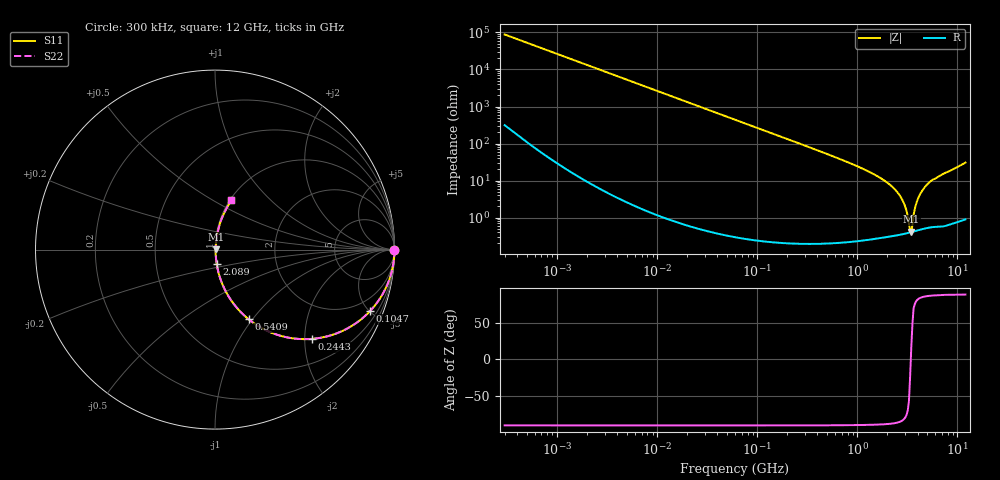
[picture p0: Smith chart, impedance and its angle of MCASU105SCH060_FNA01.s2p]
! MCASU105SCH060_FNA01  S-PARAMETER MODEL  ( Standard Model )
! Model Generated by TAIYO YUDEN Corporation (http://www.ty-top.com)
! Version 1.0
! TAIYO YUDEN Control No. 230609
! Copyright(c) 2023 TAIYO YUDEN CO.,LTD. All Rights Reserved.
! Product Description (link to TY-COMPAS)
! https://ds.yuden.co.jp/TYCOMPAS/or/detail?pn=MCASU105SCH060CFNA01&u=M
! Products Name : Multilayer Ceramic Capacitors
! Characteristics :
!  Capacitance : 6 [pF] , Rated Voltage : 50 [V] , TCC : CH / C0H
!  Case Size : 1.0 x 0.5 / 0.039 x 0.02 [mm/inch] , Thickness : 0.5 / 0.02 [mm/inch]
!  (Conditions: Temperature = 25 [degC] , DC Bias Voltage = 0 [V])
! External Node Assignments :
!  1  o---| |---o  2
! GND o---------o GND
! Frequency Range : 0.3MHz  -  12000MHz  [ 401 STEP ]
# MHZ S RI R 50
! Freq[MHz].  S11 Real  S11 Imag  S21 Real  S21 Imag  S12 Real  S12 Imag  S22 Real  S22 Imag
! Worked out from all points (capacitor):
!   401 points, 300 kHz to 12 GHz, reference 50 ohm
!   read as one part in series: C = 6 pF near 316.3 kHz
!   lowest |Z| = 417 mohm at 3.455 GHz (marker M1)
!   series resonance near 3.42 GHz, so ESL is about 360 pH
!   S11 on the Smith chart (normalised r, x): 300 kHz: open; 104.7 MHz: 1.00, -5.06; 244.3 MHz: 1.00, -2.16; 540.9 MHz: 1.00, -0.96; 2.089 GHz: 1.01, -0.16; 12 GHz: 1.02, +0.61
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0.3  1 -0.00113  5.29e-06 0.00113  5.29e-06 0.00113  1 -0.00113
1.769972  1 -0.00667  4.95e-05 0.00667  4.95e-05 0.00667  1 -0.00667
10.44266  0.9984 -0.0393  0.00156 0.0393  0.00156 0.0393  0.9984 -0.0393
60  0.9512 -0.2152  0.0488 0.2152  0.0488 0.2152  0.9512 -0.2152
104.6549  0.8649 -0.3414  0.1351 0.3414  0.1351 0.3414  0.8649 -0.3414
244.3004  0.5384 -0.4976  0.4616 0.4976  0.4616 0.4976  0.5384 -0.4976
353.9943  0.355 -0.4772  0.645 0.4772  0.645 0.4772  0.355 -0.4772
540.8523  0.187 -0.3879  0.813 0.3879  0.813 0.3879  0.187 -0.3879
1229.528  0.0362 -0.1803  0.9638 0.1803  0.9638 0.1803  0.0362 -0.1803
2088.533  0.00921 -0.0782  0.9908 0.0782  0.9908 0.0782  0.00921 -0.0782
2448.343  0.00596 -0.0518  0.994 0.0518  0.994 0.0518  0.00596 -0.0518
2795.104  0.00444 -0.0306  0.9956 0.0306  0.9956 0.0306  0.00444 -0.0306
3026.31  0.004 -0.0182  0.996 0.0182  0.996 0.0182  0.004 -0.0182
3276.641  0.0039 -0.00586  0.9961 0.00586  0.9961 0.00586  0.0039 -0.00586
3364.605  0.00394 -0.00176  0.9961 0.00176  0.9961 0.00176  0.00394 -0.00176
3454.93  0.00401 0.00108  0.996 -0.00108  0.996 -0.00108  0.00401 0.00108
3547.679  0.0041 0.00445  0.9959 -0.00445  0.9959 -0.00445  0.0041 0.00445
3841.137  0.0048 0.0215  0.9952 -0.0215  0.9952 -0.0215  0.0048 0.0215
4050.141  0.00558 0.0326  0.9944 -0.0326  0.9944 -0.0326  0.00558 0.0326
4875.354  0.0104 0.0722  0.9896 -0.0722  0.9896 -0.0722  0.0104 0.0722
6879.757  0.0248 0.1366  0.9752 -0.1366  0.9752 -0.1366  0.0248 0.1366
12000  0.0918 0.2745  0.9082 -0.2745  0.9082 -0.2745  0.0918 0.2745
